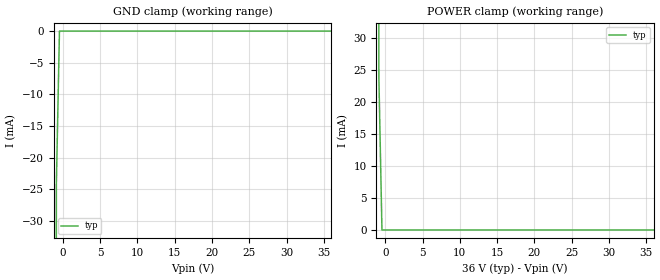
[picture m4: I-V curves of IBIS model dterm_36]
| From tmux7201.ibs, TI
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| dterm_36
[Model]   dterm_36
Model_type   Terminator
|   typ   min   max
C_comp   4.014581e-11   NA   NA
[Voltage Range]   36   NA   NA
[Temperature Range]   27   NA   NA
[Power Clamp Reference]   36   NA   NA
[GND Clamp Reference]   0   NA   NA
[GND Clamp]
|   Voltage   I(typ)   I(min)   I(max)
-5V       -11.6A     NA         NA
-1.273V   -621mA     NA         NA
-858.6mV  -24.19mA   NA         NA
-444.4mV  -30.96nA   NA         NA
36V       1.41nA     NA         NA
[POWER Clamp]
|   Voltage   I(typ)   I(min)   I(max)
-5V       13.26A     NA         NA
-1.273V   611.4mA    NA         NA
-858.6mV  23.93mA    NA         NA
-444.4mV  23.28nA    NA         NA
36V       -1.411nA   NA         NA
